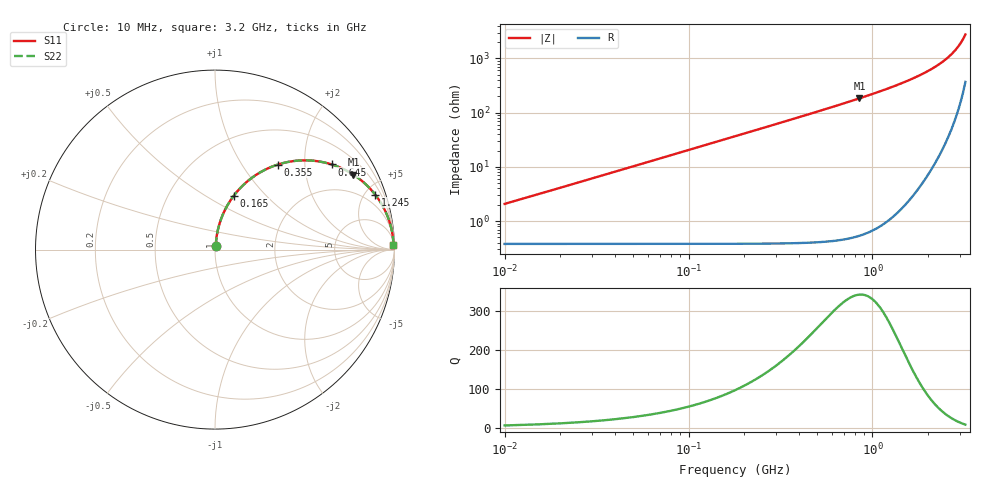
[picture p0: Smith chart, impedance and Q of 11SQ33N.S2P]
! Coilcraft 1111SQ-33N Air Core Inductor
! 14 MAR 2012
# MHZ S MA R 50
!Freq  MagS11  AngS11  MagS21  AngS21  MagS12  AngS12  MagS22  AngS22
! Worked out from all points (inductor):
!   639 points, 10 MHz to 3.2 GHz, reference 50 ohm
!   read as one part in series: L = 32.6 nH near 25 MHz
!   highest Q = 342 at 850 MHz (marker M1), where L = 34.4 nH
!   S11 on the Smith chart (normalised r, x): 10 MHz: 1.01, +0.04; 165 MHz: 1.01, +0.68; 355 MHz: 1.01, +1.47; 645 MHz: 1.01, +2.73; 1.245 GHz: 1.04, +5.81; 3.2 GHz: 14, +70
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10  0.02071 78.3  0.996 -1.2  0.996 -1.2  0.02071 78.3
20  0.04087 82.4  0.9954 -2.3  0.9954 -2.3  0.04087 82.4
30  0.0611 83.0  0.9944 -3.5  0.9944 -3.5  0.0611 83.0
40  0.08128 82.7  0.9929 -4.7  0.9929 -4.7  0.08128 82.7
50  0.1014 82.0  0.9911 -5.8  0.9911 -5.8  0.1014 82.0
65  0.1313 80.8  0.9876 -7.6  0.9876 -7.6  0.1313 80.8
85  0.1707 78.9  0.9816 -9.8  0.9816 -9.8  0.1707 78.9
105  0.2093 76.9  0.9742 -12.1  0.9742 -12.1  0.2093 76.9
165  0.3191 70.7  0.9441 -18.6  0.9441 -18.6  0.3191 70.7
250  0.4554 62.4  0.8869 -27.1  0.8869 -27.1  0.4554 62.4
355  0.5895 53.5  0.8047 -36.2  0.8047 -36.2  0.5895 53.5
440  0.6726 47.4  0.737 -42.3  0.737 -42.3  0.6726 47.4
545  0.7502 41.1  0.6585 -48.7  0.6585 -48.7  0.7502 41.1
645  0.8046 36.2  0.5912 -53.7  0.5912 -53.7  0.8046 36.2
850  0.8772 28.4  0.4776 -61.4  0.4776 -61.4  0.8772 28.4
1075  0.9224 22.4  0.3834 -67.4  0.3834 -67.4  0.9224 22.4
1245  0.9435 19.0  0.3277 -70.8  0.3277 -70.8  0.9435 19.0
1605  0.9696 13.6  0.2385 -76.1  0.2385 -76.1  0.9696 13.6
2140  0.9867 8.2  0.1483 -80.9  0.1483 -80.9  0.9867 8.2
2670  0.993 4.5  0.08498 -83.2  0.08498 -83.2  0.993 4.5
2960  0.9943 2.8  0.05682 -83.0  0.05682 -83.0  0.9943 2.8
3200  0.9946 1.6  0.03598 -80.8  0.03598 -80.8  0.9946 1.6
